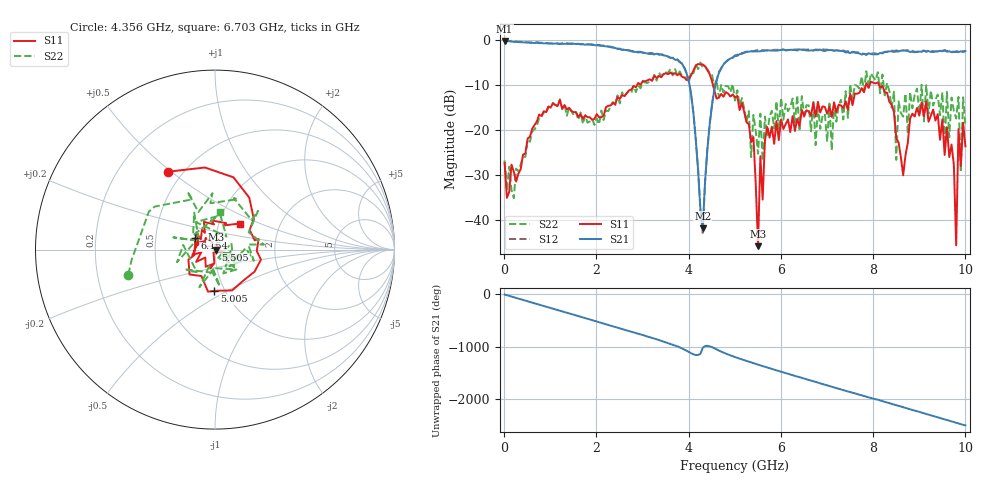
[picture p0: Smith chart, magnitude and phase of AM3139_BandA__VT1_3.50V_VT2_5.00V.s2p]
! Date/Time: Tue, Nov 13, 2018 4:57 PM
! Network Analyzer: Agilent Technologies E8364B Rev: A.07.50.67
! Sweep from 0.010 to 10.000 GHz, 201 Points, Sweep Type: LIN
! Power Supply: 3.501 V, 0.000 A
# Hz S DB R 50
!freq MagS11 AngS11 MagS21 AngS21 MagS12 AngS12 MagS22 AngS22
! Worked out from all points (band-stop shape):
!   201 points, 10 MHz to 10 GHz, reference 50 ohm
!   highest |S21| = -0.30 dB at 10 MHz (marker M1); lowest = -41.9 dB at 4.306 GHz (marker M2)
!   |S21| within 3 dB of the highest: start of sweep to 3.346 GHz; 5.092 GHz to 7.75 GHz (2.658 GHz wide, 41.4 % of centre)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
!   lowest |S11| = -45.8 dB at 5.505 GHz (marker M3), VSWR 1.01, Z = 50.5 - j0.124 ohm
!   |S11| at or under -10 dB: start of sweep to 2.886 GHz; 4.526 GHz to 7.844 GHz (3.318 GHz wide, 53.7 % of centre); 8.125 GHz to end of sweep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
!   |S22| runs from -35.2 to -5.1 dB; largest |S21 - S12| = 0.031
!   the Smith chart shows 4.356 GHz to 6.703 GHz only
!   S11 on the Smith chart (normalised r, x): 4.356 GHz: 0.42, +0.49; 5.005 GHz: 0.89, -0.43; 5.505 GHz: 1.01, -0.00; 6.154 GHz: 0.79, +0.10; 6.703 GHz: 1.25, +0.38
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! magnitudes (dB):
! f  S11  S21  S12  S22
! 10 MHz  -27.4  -0.3  -0.2  -26.8
! 1.708 GHz  -17.5  -1.0  -1.0  -18.7
! 3.357 GHz  -8.0  -3.4  -3.2  -7.3
! 4.006 GHz  -8.6  -9.3  -9.2  -9.5
! 4.306 GHz  -5.5  -41.9  -42.9  -6.1
! 4.356 GHz  -5.9  -31.5  -31.6  -6.0
! 4.555 GHz  -11.2  -11.2  -11.1  -10.3
! 5.005 GHz  -12.8  -3.6  -3.5  -13.5
! 5.405 GHz  -21.6  -2.6  -2.5  -16.7
! 5.505 GHz  -45.8  -2.6  -2.3  -25.3
! 5.554 GHz  -25.8  -2.6  -2.4  -16.4
! 6.154 GHz  -17.7  -2.3  -2.3  -15.9
! 6.703 GHz  -14.0  -2.4  -2.3  -13.6
! 8.352 GHz  -13.8  -2.6  -2.6  -11.4
! 8.501 GHz  -21.9  -2.6  -2.4  -26.7
! 8.551 GHz  -22.8  -2.6  -2.5  -13.7
! 9.55 GHz  -25.6  -2.4  -2.3  -23.4
! 9.6 GHz  -19.4  -2.7  -2.5  -11.6
! 9.8 GHz  -45.6  -2.7  -2.6  -17.5
! 9.85 GHz  -19.8  -2.8  -2.6  -12.7
! 9.9 GHz  -28.1  -2.6  -2.5  -29.4
! 10 GHz  -23.7  -2.6  -2.5  -19.1
